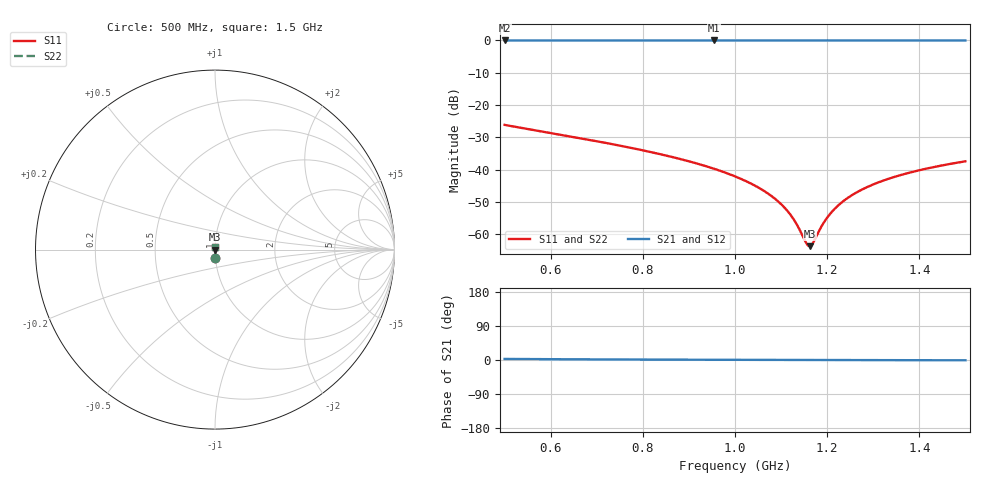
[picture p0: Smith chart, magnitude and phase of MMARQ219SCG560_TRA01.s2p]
! MMARQ219SCG560_TRA01  S-PARAMETER MODEL  ( General Type )
! Model Generated by TAIYO YUDEN Corporation (http://www.ty-top.com)
! Version 1.0
! TAIYO YUDEN Control No. 150609
! Copyright(c) 2015 TAIYO YUDEN CO.,LTD. All Rights Reserved.
! Product Description (link to TY-COMPAS)
! https://ds.yuden.co.jp/TYCOMPAS/or/detail?pn=MMARQ219SCG560JTRA01&u=M
! Products Name : Multilayer Ceramic Capacitors
! Characteristics :
!  Capacitance : 56 pF , Rated Voltage : 250V , TCC : CG / C0G
!  Case Size : 2.0 x 1.25 / 0.079 x 0.049 [mm/inch] , Thickness : 0.85 / 0.033 [mm/inch]
!  (Conditions: Temperature = 25 degC , DC Bias Current/Voltage = 0A / 0V)
! External Node Assignments :
!  1  o---| |---o  2
! GND o---------o GND
! Frequency Range : 500MHz  -  1.5GHz  [ 401 STEP ]
# MHz S RI R 50
! Freq[MHz].  S11 Real  S11 Imag  S21 Real  S21 Imag  S12 Real  S12 Imag  S22 Real  S22 Imag
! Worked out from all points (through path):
!   401 points, 500 MHz to 1.5 GHz, reference 50 ohm
!   highest |S21| = 0.00 dB at 955 MHz (marker M1); lowest = 0.0 dB at 500 MHz (marker M2)
!   lowest |S11| = -63.7 dB at 1.163 GHz (marker M3), VSWR 1.00, Z = 50.1 + j0.00194 ohm
!   |S11| at or under -10 dB: start of sweep to end of sweep
!   |S22| runs from -63.7 to -26.2 dB; largest |S21 - S12| = 0
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500  0.00274 -0.0491  0.9973 0.0491  0.9973 0.0491  0.00274 -0.0491
667.5  0.0013 -0.0303  0.9987 0.0303  0.9987 0.0303  0.0013 -0.0303
835  0.000763 -0.0175  0.9992 0.0175  0.9992 0.0175  0.000763 -0.0175
955  0.000626 -0.0103  0.9994 0.0103  0.9994 0.0103  0.000626 -0.0103
1000  0.000609 -0.00783  0.9994 0.00783  0.9994 0.00783  0.000609 -0.00783
1055  0.000606 -0.00503  0.9994 0.00503  0.9994 0.00503  0.000606 -0.00503
1077.5  0.000611 -0.00393  0.9994 0.00393  0.9994 0.00393  0.000611 -0.00393
1097.5  0.000617 -0.00297  0.9994 0.00297  0.9994 0.00297  0.000617 -0.00297
1122.5  0.000628 -0.0018  0.9994 0.0018  0.9994 0.0018  0.000628 -0.0018
1135  0.000634 -0.00122  0.9994 0.00122  0.9994 0.00122  0.000634 -0.00122
1155  0.000646 -0.000317  0.9994 0.000317  0.9994 0.000317  0.000646 -0.000317
1162.5  0.000652 1.94e-05  0.9993 -1.94e-05  0.9993 -1.94e-05  0.000652 1.94e-05
1167.5  0.000655 0.000242  0.9993 -0.000242  0.9993 -0.000242  0.000655 0.000242
1187.5  0.00067 0.00112  0.9993 -0.00112  0.9993 -0.00112  0.00067 0.00112
1197.5  0.000678 0.00156  0.9993 -0.00156  0.9993 -0.00156  0.000678 0.00156
1212.5  0.000692 0.00221  0.9993 -0.00221  0.9993 -0.00221  0.000692 0.00221
1230  0.000708 0.00295  0.9993 -0.00295  0.9993 -0.00295  0.000708 0.00295
1250  0.000728 0.00379  0.9993 -0.00379  0.9993 -0.00379  0.000728 0.00379
1275  0.000756 0.00482  0.9992 -0.00482  0.9992 -0.00482  0.000756 0.00482
1335  0.000831 0.00723  0.9992 -0.00723  0.9992 -0.00723  0.000831 0.00723
1410  0.000942 0.0101  0.9991 -0.0101  0.9991 -0.0101  0.000942 0.0101
1500  0.0011 0.0134  0.9989 -0.0134  0.9989 -0.0134  0.0011 0.0134
